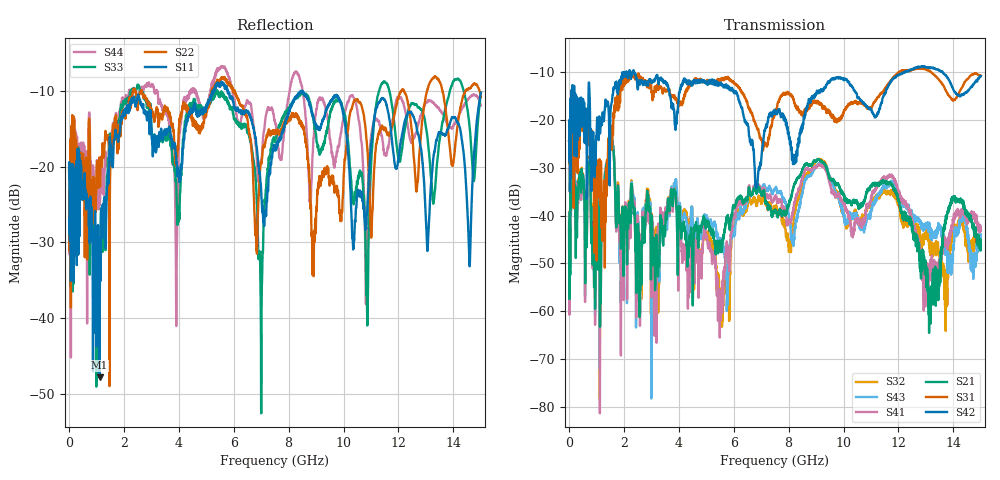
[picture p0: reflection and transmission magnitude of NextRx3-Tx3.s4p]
! FILE: N:\QM 2007\Prüfprotokolle\Highspeed\Konfektionierte Ltg\L45593-D106\D30\8216\0002\Next  Platine 1\NextRx3-Tx3.s4p
# MHz S DB R 50.00
! FREQ  S11  S12  S13  S14
!  S21  S22  S23  S24
!  S31  S32  S33  S34
!  S41  S42  S43  S44
!  DB  ANG  DB  ANG  DB  ANG  DB  ANG
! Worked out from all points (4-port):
!   2999 points, 10 MHz to 15 GHz, reference 50 ohm
!   strongest paths, dB at 10 MHz, 3.755 GHz, 7.505 GHz, 11.26 GHz, 15 GHz:
!     S42: -24.5, -16.9, -18.4, -18.8, -10.9
!     S31: -24.4, -15.2, -18.7, -15.3, -10.8
!     S21: -41.2, -35.9, -39.1, -33.3, -47.2
!     S41: -42.9, -35.1, -36.2, -33.6, -42.9
!     S43: -46.0, -34.1, -34.6, -35.9, -44.0
!     S32: -42.4, -35.1, -38.7, -36.0, -46.2
!   lowest |S11| = -47.8 dB at 1.12 GHz (marker M1), VSWR 1.01, Z = 49.7 - j0.233 ohm
!   |S11| at or under -10 dB: start of sweep to 5.249 GHz; 5.778 GHz to 8.445 GHz (2.667 GHz wide, 37.5 % of centre); 8.495 GHz to end of sweep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
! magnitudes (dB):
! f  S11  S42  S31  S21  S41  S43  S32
! 10 MHz  -19.5  -24.5  -24.4  -41.2  -42.9  -46.0  -42.4
! 1.12 GHz  -47.8  -20.7  -28.4  -47.0  -48.7  -51.2  -53.5
! 1.53 GHz  -17.3  -17.2  -23.0  -24.6  -24.5  -24.2  -24.4
! 1.89 GHz  -13.5  -12.3  -12.9  -45.3  -58.2  -58.2  -44.7
! 5.5 GHz  -9.3  -12.5  -11.5  -47.1  -61.5  -45.3  -58.2
! 6.975 GHz  -21.9  -29.0  -23.7  -35.2  -34.1  -34.1  -36.9
! 15 GHz  -10.2  -10.9  -10.8  -47.2  -42.9  -44.0  -46.2
